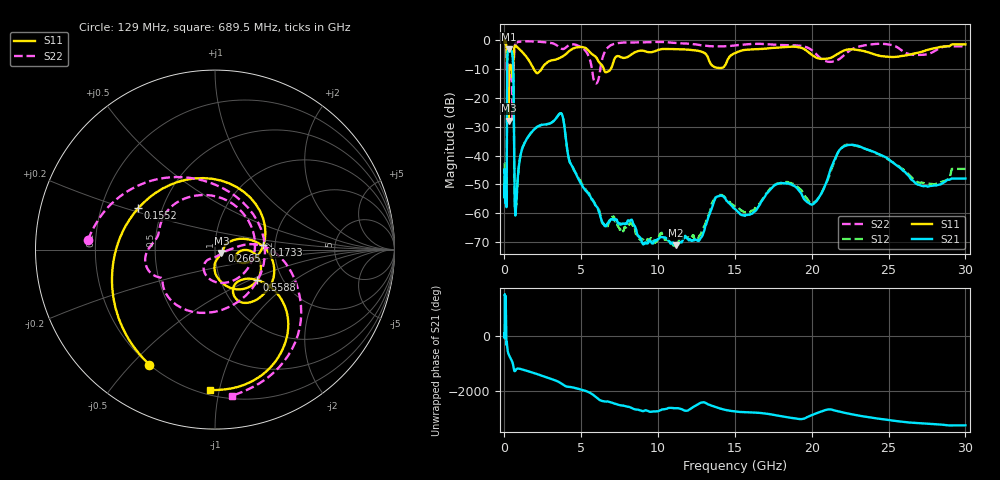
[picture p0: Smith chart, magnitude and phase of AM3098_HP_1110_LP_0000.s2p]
! Date/Time: Thu, Feb 28, 2019 8:46 AM
! Network Analyzer: Agilent Technologies E8364B Rev: A.07.50.67
! Sweep from 0.010 to 30.000 GHz, 1601 Points, Sweep Type: LOG
! Power Supply: 5.022 V, 0.002 A
# Hz S DB R 50
!freq MagS11 AngS11 MagS21 AngS21 MagS12 AngS12 MagS22 AngS22
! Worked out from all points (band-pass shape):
!   1601 points, 10 MHz to 30 GHz, reference 50 ohm
!   highest |S21| = -3.29 dB at 284.4 MHz (marker M1); lowest = -71.0 dB at 11.14 GHz (marker M2)
!   |S21| within 3 dB of the highest: 183.3 MHz to 539.1 MHz (355.8 MHz wide, 98.5 % of centre)
!   lowest |S11| = -27.9 dB at 263.8 MHz (marker M3), VSWR 1.08, Z = 53.6 - j2.02 ohm
!   |S11| at or under -10 dB: 170.1 MHz to 324.9 MHz (154.9 MHz wide, 62.6 % of centre); 1.889 GHz to 2.426 GHz (537.8 MHz wide, 24.9 % of centre); 6.46 GHz to 6.938 GHz (478.7 MHz wide, 7.15 % of centre)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
!   |S22| runs from -28.5 to -0.5 dB; largest |S21 - S12| = 0.01
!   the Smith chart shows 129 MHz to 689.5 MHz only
!   S11 on the Smith chart (normalised r, x): 129 MHz: 0.20, -0.56; 155.2 MHz: 0.37, +0.22; 173.3 MHz: 1.74, +0.09; 266.5 MHz: 1.08, -0.02; 558.8 MHz: 1.49, -0.55; 689.5 MHz: 0.23, -0.94
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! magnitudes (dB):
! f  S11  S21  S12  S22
! 10 MHz  -0.4  -45.8  -42.5  -0.5
! 38.04 MHz  -0.3  -51.3  -48.8  -0.5
! 129 MHz  -2.6  -57.6  -53.2  -3.0
! 144.7 MHz  -4.3  -51.8  -50.1  -5.8
! 155.2 MHz  -6.3  -34.2  -34.4  -10.3
! 173.3 MHz  -11.3  -10.2  -10.1  -8.5
! 225.9 MHz  -11.6  -3.9  -3.8  -8.2
! 263.8 MHz  -27.9  -3.3  -3.3  -9.6
! 266.5 MHz  -27.6  -3.3  -3.3  -9.6
! 284.4 MHz  -17.3  -3.3  -3.3  -9.6
! 550.5 MHz  -11.8  -7.2  -7.2  -27.2
! 558.8 MHz  -10.8  -8.1  -8.0  -23.9
! 689.5 MHz  -2.1  -58.8  -58.7  -1.7
! 2.084 GHz  -11.5  -30.3  -30.3  -0.7
! 3.686 GHz  -6.1  -25.4  -25.4  -3.1
! 5.959 GHz  -6.0  -57.3  -57.6  -15.1
! 7.926 GHz  -6.2  -63.5  -64.8  -1.0
! 11.14 GHz  -3.3  -71.0  -71.3  -1.1
! 14.02 GHz  -9.8  -53.9  -53.6  -2.3
! 20.1 GHz  -5.6  -56.8  -56.5  -4.1
! 22.56 GHz  -3.4  -36.3  -36.3  -3.5
! 30 GHz  -1.7  -48.0  -44.6  -2.3
